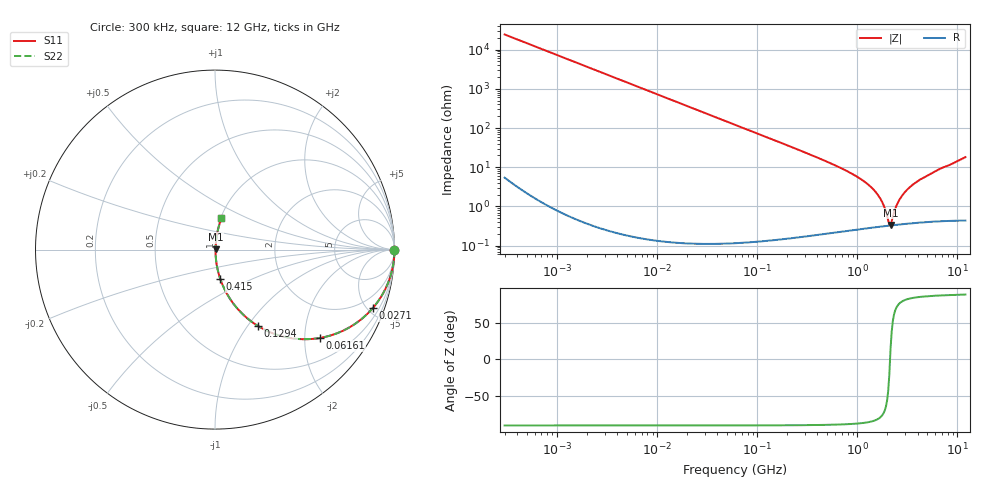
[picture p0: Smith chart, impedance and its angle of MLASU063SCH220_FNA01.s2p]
! MLASU063SCH220_FNA01  S-PARAMETER MODEL  ( General Type )
! Model Generated by TAIYO YUDEN Corporation (http://www.ty-top.com)
! Version 4.0
! TAIYO YUDEN Control No. 120810
! Copyright(c) 2009 TAIYO YUDEN CO.,LTD. All Rights Reserved.
! Product Description (link to TY-COMPAS)
! https://ds.yuden.co.jp/TYCOMPAS/or/detail?pn=MLASU063SCH220JFNA01&u=M
! Products Name : Multilayer Ceramic Capacitors
! Characteristics :
!  Capacitance : 22 pF , Rated Voltage : 50V , TCC : CH / C0H
!  Case Size : 0.6 x 0.3 / 0.024 x 0.012 [mm/inch] , Thickness : 0.3 / 0.012 [mm/inch]
!  (Conditions: Temperature = 25 degC , DC Bias Current/Voltage = 0A / 0V)
! External Node Assignments :
!  1  o---| |---o  2
! GND o---------o GND
! Frequency Range : 0.3MHz  -  12000MHz  [ 401 STEP ]
# MHz S RI R 50
! Freq[MHz].  S11 Real  S11 Imag  S21 Real  S21 Imag  S12 Real  S12 Imag  S22 Real  S22 Imag
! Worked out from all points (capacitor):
!   401 points, 300 kHz to 12 GHz, reference 50 ohm
!   read as one part in series: C = 21.9 pF near 316.3 kHz
!   lowest |Z| = 337 mohm at 2.145 GHz (marker M1)
!   series resonance near 2.122 GHz, so ESL is about 260 pH
!   S11 on the Smith chart (normalised r, x): 300 kHz: open; 27.1 MHz: 1.00, -5.37; 61.61 MHz: 1.00, -2.36; 129.4 MHz: 1.00, -1.12; 415 MHz: 1.00, -0.34; 12 GHz: 1.01, +0.36
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0.3  1 -0.00412  1.79e-05 0.00412  1.79e-05 0.00412  1 -0.00412
1.769972  0.9994 -0.0243  0.000593 0.0243  0.000593 0.0243  0.9994 -0.0243
10.44266  0.9798 -0.1405  0.0202 0.1405  0.0202 0.1405  0.9798 -0.1405
27.10171  0.8782 -0.3268  0.1218 0.3268  0.1218 0.3268  0.8782 -0.3268
60  0.5952 -0.4904  0.4048 0.4904  0.4048 0.4904  0.5952 -0.4904
61.61074  0.5823 -0.4927  0.4177 0.4927  0.4177 0.4927  0.5823 -0.4927
129.3602  0.2398 -0.4258  0.7602 0.4258  0.7602 0.4258  0.2398 -0.4258
202.9496  0.1133 -0.3148  0.8867 0.3148  0.8867 0.3148  0.1133 -0.3148
353.9943  0.0401 -0.1916  0.9599 0.1916  0.9599 0.1916  0.0401 -0.1916
414.98  0.0294 -0.1635  0.9706 0.1635  0.9706 0.1635  0.0294 -0.1635
848.5281  0.00756 -0.0714  0.9924 0.0714  0.9924 0.0714  0.00756 -0.0714
1331.232  0.00391 -0.033  0.9961 0.033  0.9961 0.033  0.00391 -0.033
1560.575  0.00342 -0.0213  0.9966 0.0213  0.9966 0.0213  0.00342 -0.0213
1735.023  0.00326 -0.0139  0.9967 0.0139  0.9967 0.0139  0.00326 -0.0139
2088.533  0.00324 -0.00117  0.9968 0.00117  0.9968 0.00117  0.00324 -0.00117
2144.601  0.00326 0.000813  0.9967 -0.000813  0.9967 -0.000813  0.00326 0.000813
2202.174  0.00329 0.00251  0.9967 -0.00251  0.9967 -0.00251  0.00329 0.00251
2448.343  0.00347 0.00955  0.9965 -0.00955  0.9965 -0.00955  0.00347 0.00955
2650.866  0.00368 0.0148  0.9963 -0.0148  0.9963 -0.0148  0.00368 0.0148
3454.93  0.00478 0.0329  0.9952 -0.0329  0.9952 -0.0329  0.00478 0.0329
5868.704  0.00982 0.0753  0.9902 -0.0753  0.9902 -0.0753  0.00982 0.0753
12000  0.0356 0.1736  0.9644 -0.1736  0.9644 -0.1736  0.0356 0.1736
